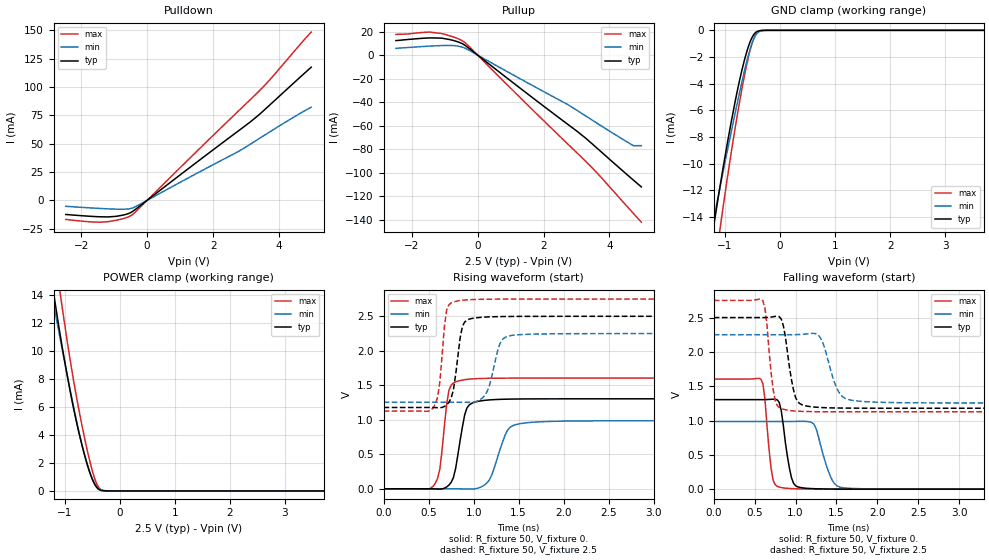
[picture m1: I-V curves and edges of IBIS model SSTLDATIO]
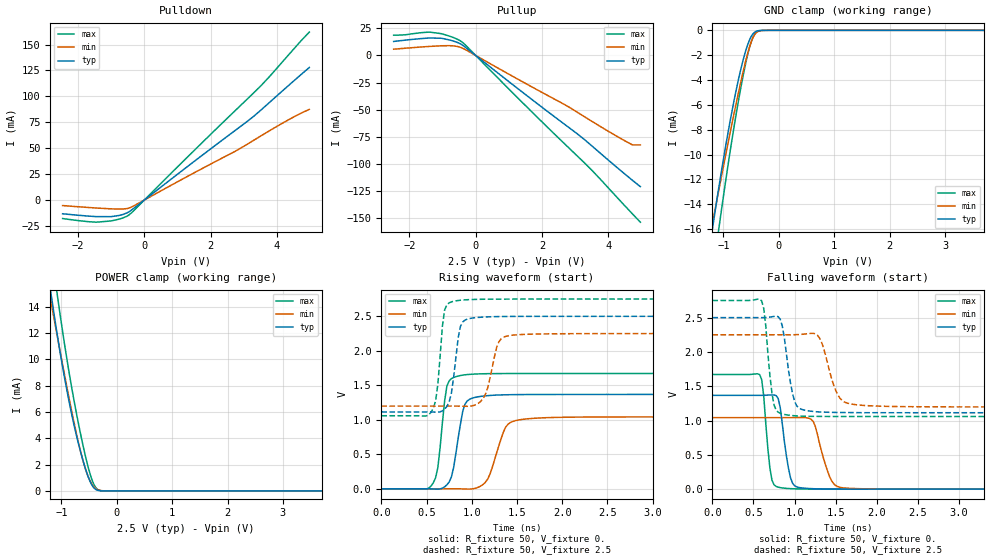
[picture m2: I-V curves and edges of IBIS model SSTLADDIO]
|   Signal Integrity Software, INC.
|   IBIS Model for IBIS QUALITY EXAMPLE
|Copyright Signal Integrity Software, Inc. Tue Nov 11 10:11:37 2003
|IV and VT curves generated from SiAuditor Spice to IBIS 5.1.1
[IBIS Ver]   3.2
[Disclaimer] THESE DESIGNS ARE PROVIDED "AS IS" WITH NO
   WARRANTY WHATSOEVER AND SIGNAL INTEGRITY SOFTWARE
   SPECIFICALLY DISCLAIMS ANY IMPLIED WARRANTIES OF
   MERCHANTABILITY, FITNESS FOR A PARTICULAR PURPOSE,
   OR AGAINST INFRINGEMENT.
[File Name]  iq_example.ibs
[File Rev]   1.0
[Date]   3/30/2004
[Source]   Developed by:
   Signal Integrity Software, Inc.
   6 Clock Tower Place, Suite 250
   Maynard, MA 01754
   support@sisoft.com
[Notes]
   Revision History
   Rev 1.0
   - 03/30/04 Release as iq_example. RJH
   IBIS Quality Notes
|IQ SUMMARY Overall Quality of component and models Level 2
|IQ Level 0 - 0 errors 12 warnings
|IQ Level 1 - All checks done for completeness and correctness
|IQ Level 2 - HSPICE Coorelation (2003.09) completed FOM =99%
|IQ Buffer SSTLDATIO/SSTLADDIO:   Quality level 2
|IQ Level 0
|   All I/O Models: When running through ibischk3, this file
|   contains 12 warnings about pullup and pulldown being non-monotonic.
|   This is due to an IBIS Parser Bug, BUG71.
| IQ WARNING (line  209) - Pulldown Maximum data is non-monotonic
| IQ WARNING (line  210) - Pulldown Typical data is non-monotonic
|   IBISHCK 4.0 produces 0 errors and 0 warnings
|IQ Level 1
|   All Level 1 checks performed and are either OK or NA
|   Limitations: Ccomp is a compromise between driving and receiving.
|IQ Level 2
|   Using VT IBIS Data compared to source hspice models FOM = 99%.
|IQ BEGIN IBIS Quality Checklist
|IQ FILE: iq_example.ibs   IQ Level:   2
|IQ XX  2.1   LEVEL 0  Header passes IBISCHK
|IQ XX  2.2   LEVEL 0  Latest [IBIS ver] used
|IQ XX  2.3   LEVEL 0  Do not use [Comment Char]
|IQ XX  2.4   LEVEL 0  [File Name] is correct
|IQ XX  2.5   LEVEL 0  [File Rev] is correct
|IQ XX  2.6   LEVEL 0  [Date] is correct
|IQ XX  2.7   LEVEL 0  [Source] is complete
|IQ XX  2.8   LEVEL 0  [Notes] is complete
|IQ XX  2.9   OPTIONAL [Disclaimer] and [Copyright]
|IQ COMPONENT: IQ_EXAMPLE   IQ Level:   2
|IQ XX  3.1.1   LEVEL 0  [Package] must have typical values
|IQ XX  3.1.2   LEVEL 0  [Package] Parasitics must be reasonable
|IQ XX  3.1.3   LEVEL 0  [Define Package Model] present if [Package Model] is p
|IQ XX  3.1.4   LEVEL 1  [Package] parasitics are validated against data sheet
|IQ XX  3.2.1   LEVEL 0  [Pin] section complete
|IQ XX  3.2.2   LEVEL 0  [Pin] model names not too long
|IQ XX  3.2.3   LEVEL 0  [Pin] models present in file
|IQ XX  3.2.4   OPTIONAL [Pin] RLC complete
|IQ XX  3.2.5   LEVEL 1  [Pin] RLC parasitics are validated against data sheet
|IQ NA  3.3.1   LEVEL 0  [Diff Pin] referenced pins exist
|IQ NA  3.3.2   LEVEL 0  [Diff Pin] Vdiff and Tskew complete and reasonable
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Pinlist data from example.doc Document #: ABC123, Revision 0.10
SPICE MODELS Release 1.0 XYZ 7/1/03
PDF specifications dated 4/20/03 from EFG345
Package Parameter are from  package_electrical_model.pdf
[Copyright]   Copyright 2002, Signal Integrity Software, Inc.,
   All Rights Reserved
[Component] IQ_EXAMPLE
[Manufacturer] ABC
[Package]
R_pkg 856m   NA   NA
L_pkg 6.706nH NA   NA
C_pkg 2.681pF NA   NA
[Pin]   signal_name   model_name   R_pin L_pin C_pin
|Ball   Pad Name   CellName
U10   RX_A[0]   SSTLDATIO
T9   RX_A[1]   SSTLDATIO
T10   RX_A[2]   SSTLDATIO
R10   RX_A[3]   SSTLDATIO
P9   RX_A[4]   SSTLDATIO
P10   RX_A[5]   SSTLDATIO
N8   RX_A[6]   SSTLDATIO
N10   RX_A[7]   SSTLDATIO
M9   RX_A[8]   SSTLDATIO
M10   RX_A[9]   SSTLDATIO
L8   RX_CLK_A   SSTLDATIO
T6   TX_A[0]   SSTLADDIO
T8   TX_A[1]   SSTLADDIO
R7   TX_A[2]   SSTLADDIO
R8   TX_A[3]   SSTLADDIO
P8   TX_A[4]   SSTLADDIO
N6   TX_A[5]   SSTLADDIO
N7   TX_A[6]   SSTLADDIO
M6   TX_A[7]   SSTLADDIO
M8   TX_A[8]   SSTLADDIO
L6   TX_A[9]   SSTLADDIO
AF4   TX_CLK_A   SSTLADDIO
AW35   VDD   POWER
AW33   VDD   POWER
AV37   VDD   POWER
AV34   VDD   POWER
AU33   VDD   POWER
AT37   VDD   POWER
AT34   VDD   POWER
AT31   VDD   POWER
AR39   VDD   POWER
AP37   VDD   POWER
AP34   VDD   POWER
AP31   VDD   POWER
AL39   VDD   POWER
AL33   VDD   POWER
AK37   VDD   POWER
AK30   VDD   POWER
AK29   VDD   POWER
AJ31   VDD   POWER
AF30   VDD   POWER
W27   VSS   GND
W26   VSS   GND
V27   VSS   GND
V26   VSS   GND
V25   VSS   GND
V24   VSS   GND
V23   VSS   GND
V22   VSS   GND
V21   VSS   GND
| Models and submodels in the file (2): SSTLDATIO (I/O), SSTLADDIO (I/O)
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|   MODEL SSTLDATIO
[Model]   SSTLDATIO
Model_type  I/O
Polarity   Non-Inverting
Enable   Active-Low
|C_comp_off 3.21p   3.19p  3.26p
|C_comp_on  579.10f 586.9f 612.07f
C_comp 1.896p 1.891p 1.939p
|SiSoft Rth_r 45.85 64.07 35.71
|SiSoft Rth_f 44.63 63.09 34.74
|SiSoft Rth_i 174.57e6 62.85e6 192.30e6
Cref  = 5.0pF
Vmeas = 1.25V
Vinh  = 1.6V
Vinl  = 0.9V
[Model Spec]
S_overshoot_high   2.8  2.55 3.05
S_overshoot_low   -0.3 -0.3 -0.3
|Sisoft Overshoot_High   3.0  NA   NA
|SiSoft AC_Overshoot_High   2.8  NA   NA
|SiSoft AC_Overshoot_Time   0.5ns
|SiSoft Vin_AC_High   1.60 NA   NA
|SiSoft Vin_DC_High   1.39 NA   NA
|SiSoft Vmeas   1.25 NA   NA
|SiSoft Vin_Meas_High   1.25 NA   NA
|SiSoft Vin_Meas_Low   1.25 NA   NA
|SiSoft Vin_DC_Low   1.11 NA   NA
|SiSoft Vin_AC_Low   0.90 NA   NA
|SiSoft AC_Overshoot_Low   -0.3 NA   NA
|Sisoft Overshoot_Low   -0.5 NA   NA
|SiSoft Vmeas_time   1.5nS
|SiSoft Non_monotonic_time 0.1ns NA NA
|SiSoft Vmeas_time 1.5nS
[Temperature Range]   25   125   0
||SiSoft hspice models definitions:
|SiSoft Corevdd = 1.5V
|SiSoft Hspice ff   sstldatio_wrappers.mod sstldat_ff
|SiSoft Hspice tt   sstldatio_wrappers.mod sstldat_tt
|SiSoft Hspice ss   sstldatio_wrappers.mod sstldat_ss
[Voltage Range] 2.5 2.25 2.75
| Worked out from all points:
|   slope of the pulldown table from 0 to 0.375 V, typ, clamps not added: 44.4 ohm
|   slope of the pullup table from 0 to 0.375 V, typ, clamps not added: 45.5 ohm
|   GND clamp passes 1 mA (typ) near -0.55 V on its own axis
|   POWER clamp passes 1 mA (typ) near -0.51 V on its own axis
|   rising waveform, R_fixture 50, V_fixture 0.: 20-80 % time 103ps typ, 154ps min, 80.1ps max; typ from 0 V to 1.3 V
|   rising waveform, R_fixture 50, V_fixture 2.5: 20-80 % time 81.2ps typ, 114ps min, 69.3ps max; typ from 1.18 V to 2.5 V
|   falling waveform, R_fixture 50, V_fixture 0.: 20-80 % time 96.1ps typ, 148ps min, 71.6ps max; typ from 1.3 V to 0 V
|   falling waveform, R_fixture 50, V_fixture 2.5: 20-80 % time 102ps typ, 155ps min, 79.2ps max; typ from 2.5 V to 1.18 V
[Pulldown]
-2.467V   -12.49mA   -5.286mA   -16.85mA
-1.414V   -14.56mA   -7.199mA   -19.31mA
-931.8mV  -14.12mA   -7.807mA   -17.6mA
-691mV    -12.83mA   -7.838mA   -15.91mA
-450.1mV  -9.967mA   -6.856mA   -12.64mA
2.734V    60.57mA    42.62mA    77.88mA
3.14V     69.49mA    49.75mA    89.21mA
3.531V    79.17mA    56.98mA    100.5mA
4.977V    117.6mA    82.25mA    148.6mA
[Pullup]
-2.477V   12.27mA    5.699mA    17.55mA
-1.453V   14.59mA    7.604mA    19.52mA
-1.092V   14.39mA    8.078mA    18.29mA
-610mV    11.36mA    7.732mA    14.12mA
-369.1mV  8.042mA    5.691mA    10.23mA
2.657V    -57.2mA    -40.84mA   -73.48mA
3.04V     -65.26mA   -47.45mA   -83.79mA
3.522V    -76.61mA   -56.1mA    -97.12mA
4.726V    -106.3mA   -77.02mA   -134.6mA
4.967V    -112.1mA   -77.02mA   -142mA
[GND Clamp]
-2.467V   -51.3mA    -41.4mA    -64.01mA
-1.259V   -16.26mA   -15.4mA    -20.15mA
-1.184V   -14.23mA   -13.81mA   -17.8mA
-1.108V   -12.26mA   -12.23mA   -15.53mA
-1.033V   -10.36mA   -10.67mA   -13.32mA
-881.6mV  -6.831mA   -7.589mA   -9.116mA
-692.8mV  -3.051mA   -3.938mA   -4.477mA
-541.8mV  -875.3uA   -1.435mA   -1.517mA
-475.7mV  -327.9uA   -646.9uA   -645.5uA
-409.6mV  -81.29uA   -199.4uA   -177.9uA
-211.4mV  -214.9nA   -1.565uA   -363nA
4.977V    0A         0A         0A
[Power Clamp]
-2.467V   51.63mA    40.88mA    54.54mA
-1.253V   15.57mA    14.49mA    19.17mA
-1.177V   13.56mA    12.89mA    16.88mA
-1.101V   11.66mA    11.31mA    14.71mA
-1.026V   9.866mA    9.749mA    12.62mA
-873.7mV  6.618mA    6.719mA    8.749mA
-684mV    3.274mA    3.279mA    4.677mA
-589.2mV  1.918mA    1.873mA    2.92mA
-494.3mV  820.8uA    838.9uA    1.413mA
-427.9mV  310.8uA    379.8uA    620.8uA
-361.5mV  73.56uA    131.1uA    169.6uA
4.967V    0A         0A         0A
[Ramp]
dV/dt_r .783/100.737p .592/153.122p .963/77.797p
dV/dt_f .793/101.791p .597/154.063p .974/78.215p
[Rising Waveform]
R_fixture = 50
V_fixture = 0.
0s        0V         4.622uV    9.665uV
575ps     -1.769mV   172.3nV    83mV
625ps     -4.706mV   6.887uV    293.2mV
725ps     53.94mV    95.13uV    1.428V
900ps     1.069V     -1.756mV   1.582V
1.025ns   1.26V      2.849mV    1.596V
1.175ns   1.288V     130.6mV    1.602V
1.4ns     1.3V       884.9mV    1.604V
1.825ns   1.304V     975.5mV    1.605V
25ns      1.304V     986.2mV    1.605V
[Rising Waveform]
R_fixture = 50
V_fixture = 2.5
V_fixture_min = 2.25
V_fixture_max = 2.75
0s        1.179V     1.255V     1.127V
550ps     1.178V     1.255V     1.174V
625ps     1.175V     1.255V     1.554V
700ps     1.216V     1.255V     2.591V
875ps     2.353V     1.255V     2.733V
950ps     2.459V     1.253V     2.74V
1.15ns    2.49V      1.41V      2.748V
1.325ns   2.497V     2.172V     2.749V
1.625ns   2.499V     2.24V      2.75V
25ns      2.5V       2.25V      2.75V
[Falling Waveform]
R_fixture = 50
V_fixture = 0.
0s        1.304V     986.2mV    1.605V
575ps     1.304V     986.2mV    1.604V
625ps     1.304V     986.2mV    1.318V
725ps     1.31V      986.2mV    134.4mV
825ps     1.144V     986.1mV    23.28mV
950ps     165.2mV    986.2mV    8.106mV
1.225ns   6.943mV    945mV      1.424mV
1.45ns    1.837mV    124.9mV    461.4uV
1.75ns    442.9uV    8.29mV     122.7uV
25ns      0V         4.624uV    9.665uV
[Falling Waveform]
R_fixture = 50
V_fixture = 2.5
V_fixture_min = 2.25
V_fixture_max = 2.75
0s        2.5V       2.25V      2.75V
600ps     2.5V       2.25V      2.743V
650ps     2.501V     2.25V      2.396V
725ps     2.511V     2.25V      1.459V
800ps     2.513V     2.25V      1.19V
1.025ns   1.277V     2.252V     1.136V
1.3ns     1.19V      2.211V     1.128V
1.575ns   1.182V     1.347V     1.127V
2ns       1.179V     1.267V     1.127V
25ns      1.179V     1.255V     1.127V
|   MODEL SSTLADDIO
[Model]   SSTLADDIO
Model_type  I/O
Polarity   Non-Inverting
Enable   Active-Low
|C_comp_off 3.235p 3.202p 3.287p
|C_comp_on 619.288f 612.477f 653.411f
C_comp 1.927p 1.907p 1.97p
|SiSoft Rth_r 41.45   57.98   32.32
|SiSoft Rth_f 40.22   57.02   31.34
|SiSoft Rth_i 174.88e6 62.08e6 188.23e6
Cref = 0.1pF
Vmeas = 1.25V
Vinh = 1.6V
Vinl = 0.9V
[Model Spec]
S_overshoot_high   2.8  2.55 3.05
S_overshoot_low   -0.3 -0.3 -0.3
|Sisoft Overshoot_High   3.0  NA   NA
|SiSoft AC_Overshoot_High   2.8  NA   NA
|SiSoft AC_Overshoot_Time   0.5ns
|SiSoft Vin_AC_High   1.60 NA   NA
|SiSoft Vin_DC_High   1.39 NA   NA
|SiSoft VmeasR   1.25 NA   NA
|SiSoft VmeasF   1.25 NA   NA
|SiSoft Vin_Meas_High   1.25 NA   NA
|SiSoft Vin_Meas_Low   1.25 NA   NA
|SiSoft Vin_DC_Low   1.11 NA   NA
|SiSoft Vin_AC_Low   0.90 NA   NA
|SiSoft AC_Overshoot_Low   -0.3 NA   NA
|Sisoft Overshoot_Low   -0.5 NA   NA
|SiSoft Vmeas_time   1.5nS
[Temperature Range]   25   125   0
||SiSoft hspice models definitions:
|SiSoft Corevdd = 1.2V
|SiSoft Hspice ff   sstladdio_wrappers.mod sstladd_ff
|SiSoft Hspice tt   sstladdio_wrappers.mod sstladd_tt
|SiSoft Hspice ss   sstladdio_wrappers.mod sstladd_ss
[Voltage Range] 2.5 2.25 2.75
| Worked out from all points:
|   slope of the pulldown table from 0 to 0.375 V, typ, clamps not added: 39.9 ohm
|   slope of the pullup table from 0 to 0.375 V, typ, clamps not added: 41.1 ohm
|   GND clamp passes 1 mA (typ) near -0.55 V on its own axis
|   POWER clamp passes 1 mA (typ) near -0.51 V on its own axis
|   rising waveform, R_fixture 50, V_fixture 0.: 20-80 % time 103ps typ, 154ps min, 79.9ps max; typ from 0 V to 1.37 V
|   rising waveform, R_fixture 50, V_fixture 2.5: 20-80 % time 79.6ps typ, 112ps min, 68.2ps max; typ from 1.11 V to 2.5 V
|   falling waveform, R_fixture 50, V_fixture 0.: 20-80 % time 95.6ps typ, 148ps min, 71.2ps max; typ from 1.37 V to 0 V
|   falling waveform, R_fixture 50, V_fixture 2.5: 20-80 % time 102ps typ, 156ps min, 78.7ps max; typ from 2.5 V to 1.11 V
[Pulldown]
-2.465V   -13.29mA   -5.35mA    -17.89mA
-1.45V    -16.02mA   -7.73mA    -21.41mA
-1.006V   -16.07mA   -8.53mA    -20.22mA
-644.8mV  -13.94mA   -8.665mA   -17.3mA
-464.3mV  -11.38mA   -7.784mA   -14.4mA
2.748V    67.36mA    47.18mA    86.55mA
3.53V     87.23mA    62.19mA    110.8mA
4.493V    114.6mA    79.98mA    145.3mA
4.974V    127.9mA    87.5mA     162.1mA
[Pullup]
-2.474V   12.95mA    5.797mA    18.73mA
-2.113V   14.19mA    6.709mA    19.15mA
-1.391V   16.15mA    8.365mA    21.6mA
-1.03V    15.87mA    8.96mA     20.1mA
-669.1mV  13.28mA    8.846mA    16.52mA
-428.4mV  10.15mA    7.128mA    12.78mA
1.618V    -38.87mA   -27.77mA   -49.86mA
3.039V    -71.85mA   -52.01mA   -92.18mA
3.521V    -84.04mA   -61.18mA   -106.6mA
4.484V    -109.2mA   -78.63mA   -138.5mA
4.725V    -115.3mA   -82.61mA   -146.3mA
4.965V    -121.2mA   -82.61mA   -154mA
[GND Clamp]
-2.465V   -56.53mA   -45.59mA   -70.57mA
-1.257V   -17.73mA   -16.88mA   -21.8mA
-1.182V   -15.48mA   -15.13mA   -19.2mA
-1.106V   -13.29mA   -13.38mA   -16.7mA
-1.031V   -11.19mA   -11.66mA   -14.3mA
-879.9mV  -7.313mA   -8.264mA   -9.757mA
-691.2mV  -3.224mA   -4.243mA   -4.745mA
-540.2mV  -896.2uA   -1.503mA   -1.566mA
-474.2mV  -326.4uA   -659uA     -650.4uA
-408.1mV  -79.03uA   -196.6uA   -174.1uA
-209.9mV  -204.9nA   -1.507uA   -344.2nA
4.974V    0A         0A         0A
[Power Clamp]
-2.465V   56.74mA    44.98mA    59.91mA
-1.252V   16.92mA    15.88mA    20.63mA
-1.176V   14.68mA    14.12mA    18.08mA
-1.1V     12.56mA    12.38mA    15.7mA
-1.025V   10.58mA    10.65mA    13.45mA
-873mV    7.052mA    7.313mA    9.316mA
-683.5mV  3.468mA    3.526mA    4.955mA
-588.7mV  2.016mA    1.989mA    3.075mA
-512.9mV  1.051mA    1.058mA    1.76mA
-437mV    374uA      443.6uA    734.9uA
-361.2mV  73.47uA    132.1uA    170.6uA
4.965V    0A         0A         0A
[Ramp]
dV/dt_r .821/100.787p .625/153.246p 1.003/77.346p
dV/dt_f .832/101.869p .631/154.367p 1.015/77.799p
[Rising Waveform]
R_fixture = 50
V_fixture = 0.
0s        0V         5.102uV    10.43uV
575ps     -1.881mV   114.5nV    87.44mV
625ps     -4.931mV   7.621uV    307.8mV
725ps     57.28mV    101.8uV    1.489V
900ps     1.123V     -1.88mV    1.648V
1.025ns   1.321V     3.142mV    1.662V
1.175ns   1.35V      138.4mV    1.668V
1.4ns     1.363V     934.6mV    1.67V
1.825ns   1.367V     1.031V     1.671V
25ns      1.367V     1.042V     1.671V
[Rising Waveform]
R_fixture = 50
V_fixture = 2.5
V_fixture_min = 2.25
V_fixture_max = 2.75
0s        1.114V     1.198V     1.059V
550ps     1.113V     1.198V     1.109V
625ps     1.11V      1.198V     1.514V
700ps     1.154V     1.198V     2.592V
875ps     2.355V     1.198V     2.733V
950ps     2.459V     1.196V     2.741V
1.15ns    2.49V      1.368V     2.748V
1.325ns   2.497V     2.173V     2.749V
1.6ns     2.499V     2.239V     2.75V
25ns      2.5V       2.25V      2.75V
[Falling Waveform]
R_fixture = 50
V_fixture = 0.
0s        1.367V     1.042V     1.671V
575ps     1.367V     1.042V     1.669V
625ps     1.368V     1.042V     1.356V
725ps     1.373V     1.042V     131.3mV
825ps     1.191V     1.042V     22.81mV
925ps     307.3mV    1.042V     9.422mV
1.225ns   6.745mV    988.9mV    1.372mV
1.45ns    1.789mV    122.1mV    449.4uV
1.725ns   485.6uV    9.234mV    133.5uV
25ns      0V         5.102uV    10.43uV
[Falling Waveform]
R_fixture = 50
V_fixture = 2.5
V_fixture_min = 2.25
V_fixture_max = 2.75
0s        2.5V       2.25V      2.75V
600ps     2.5V       2.25V      2.742V
725ps     2.512V     2.25V      1.397V
800ps     2.514V     2.25V      1.122V
975ps     1.393V     2.25V      1.072V
1.05ns    1.185V     2.254V     1.066V
1.3ns     1.126V     2.209V     1.06V
1.575ns   1.117V     1.296V     1.059V
2ns       1.114V     1.211V     1.059V
25ns      1.114V     1.198V     1.059V
